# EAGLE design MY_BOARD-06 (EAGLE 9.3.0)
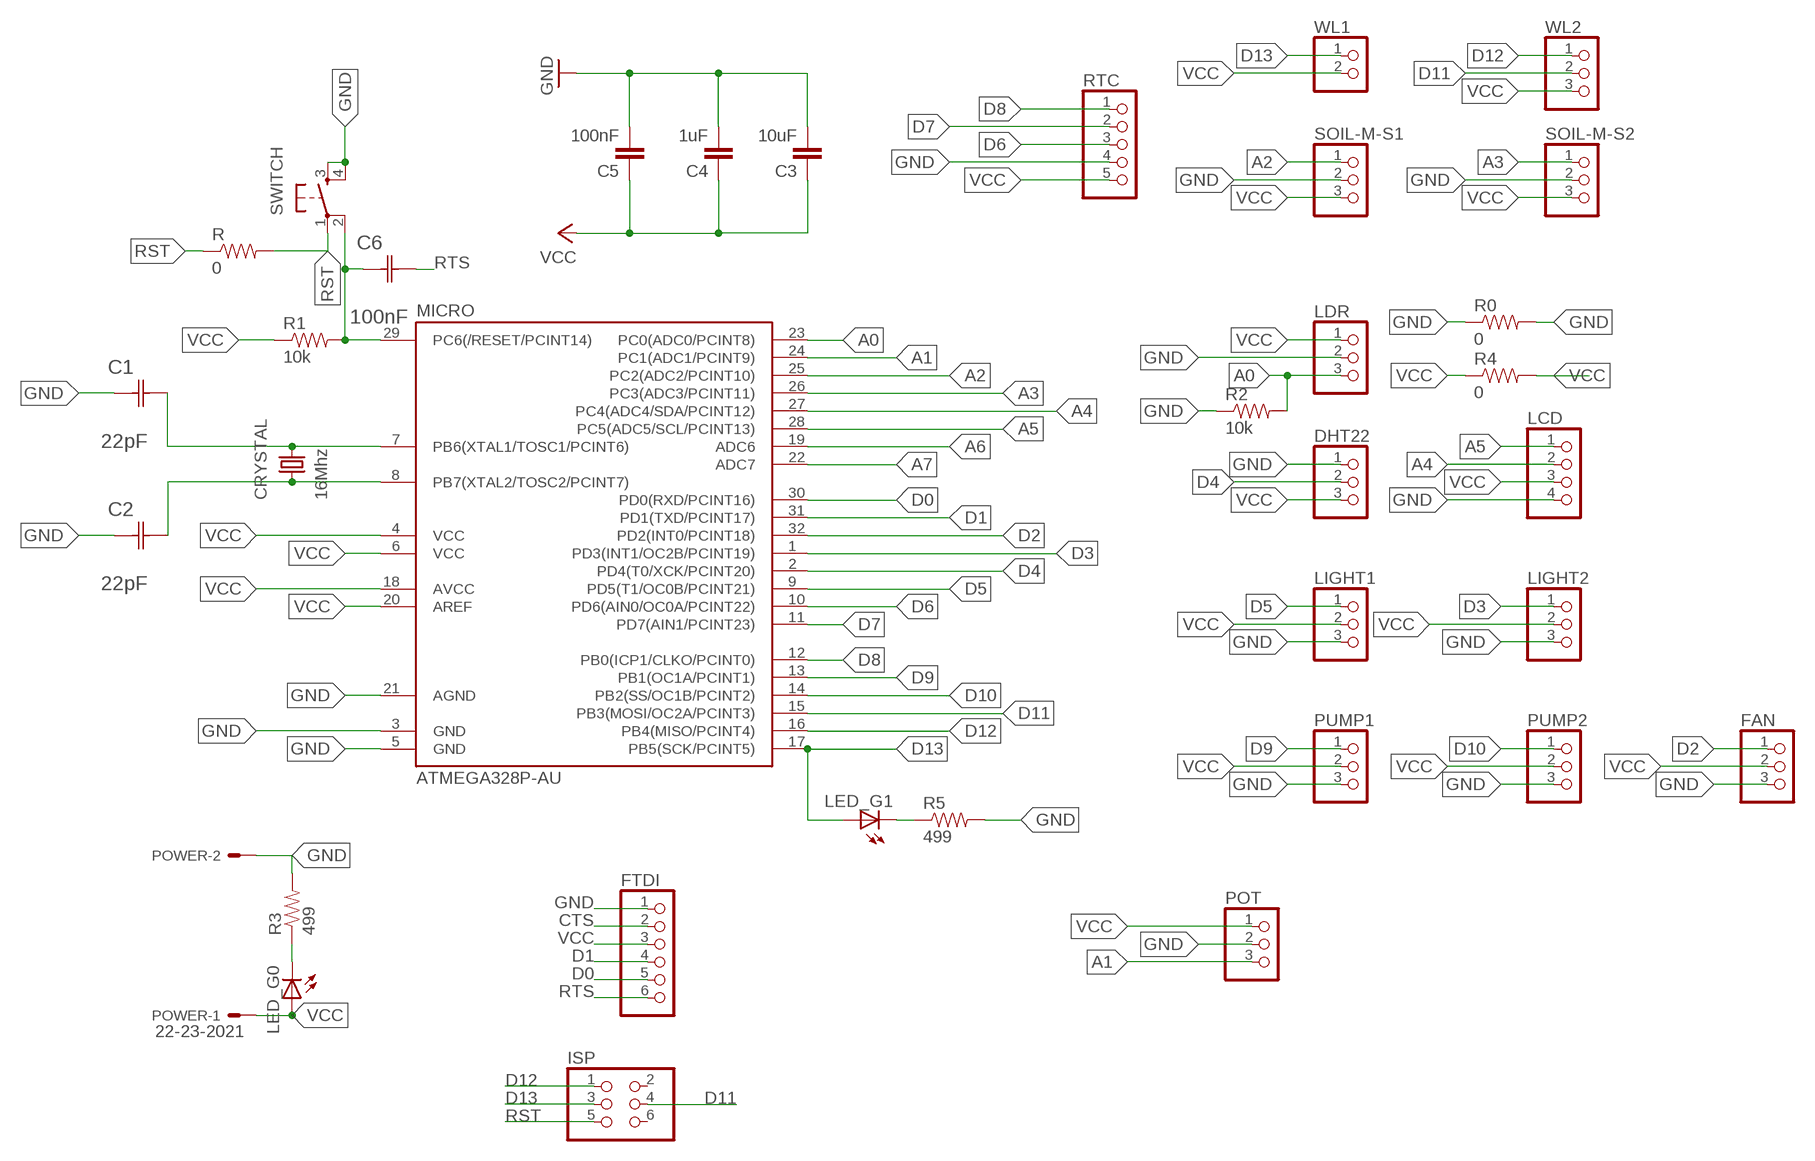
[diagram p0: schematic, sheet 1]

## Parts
C1  22pF  0612ZC225MAT2A  [CAPC3216X178N]
C2  22pF  0612ZC225MAT2A  [CAPC3216X178N]
C3  10uF  CAP1206  [1206]
C4  1uF  CAP1206  [1206]
C5  100nF  CAP1206  [1206]
C6  100nF  0612ZC225MAT2A  [CAPC3216X178N]
CRYSTAL  16Mhz  CSM-7X-DU  [CSM-7X-DU]
DHT22  PINHD-1X3/90  [1X03/90]
FAN  PINHD-1X3/90  [1X03/90]
FTDI  PINHD-1X6  [1X06]
ISP  PINHD-2X3-SMD  [2X03SMD]
LCD  PINHD-1X4/90  [1X04/90]
LDR  PINHD-1X3/90  [1X03/90]
LED_G0  LED1206  [1206]
LED_G1  LED1206  [1206]
LIGHT1  PINHD-1X3/90  [1X03/90]
LIGHT2  PINHD-1X3/90  [1X03/90]
MICRO  ATMEGA328P-AU  ATMEGA48/88/168-AU  [TQFP32-08]
POT  PINHD-1X3  [1X03]
POWER  22-23-2021  [22-23-2021]
PUMP1  PINHD-1X3/90  [1X03/90]
PUMP2  PINHD-1X3/90  [1X03/90]
R  0  RESISTOR1206  [1206]
R0  0  RESISTOR1206  [1206]
R1  10k  RESISTOR1206  [1206]
R2  10k  RESISTOR1206  [1206]
R3  499  RESISTOR1206  [1206]
R4  0  RESISTOR1206  [1206]
R5  499  RESISTOR1206  [1206]
RTC  PINHD-1X5/90  [1X05/90]
SOIL-M-S1  PINHD-1X3/90  [1X03/90]
SOIL-M-S2  PINHD-1X3/90  [1X03/90]
SWITCH  6MM_SWITCH6MM_SWITCH  [6MM_SWITCH]
WL1  PINHD-1X2/90  [1X02/90]
WL2  PINHD-1X3/90  [1X03/90]

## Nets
A0: LDR.3 MICRO.23(PC0(ADC0/PCINT8)) R2.2
A1: MICRO.24(PC1(ADC1/PCINT9)) POT.3
A2: MICRO.25(PC2(ADC2/PCINT10)) SOIL-M-S1.1
A3: MICRO.26(PC3(ADC3/PCINT11)) SOIL-M-S2.1
A4: LCD.2 MICRO.27(PC4(ADC4/SDA/PCINT12))
A5: LCD.1 MICRO.28(PC5(ADC5/SCL/PCINT13))
A6: MICRO.19(ADC6)
A7: MICRO.22(ADC7)
CTS: FTDI.2
D0: FTDI.5 MICRO.30(PD0(RXD/PCINT16))
D1: FTDI.4 MICRO.31(PD1(TXD/PCINT17))
D2: FAN.1 MICRO.32(PD2(INT0/PCINT18))
D3: LIGHT2.1 MICRO.1(PD3(INT1/OC2B/PCINT19))
D4: DHT22.2 MICRO.2(PD4(T0/XCK/PCINT20))
D5: LIGHT1.1 MICRO.9(PD5(T1/OC0B/PCINT21))
D6: MICRO.10(PD6(AIN0/OC0A/PCINT22)) RTC.3
D7: MICRO.11(PD7(AIN1/PCINT23)) RTC.2
D8: MICRO.12(PB0(ICP1/CLKO/PCINT0)) RTC.1
D9: MICRO.13(PB1(OC1A/PCINT1)) PUMP1.1
D10: MICRO.14(PB2(SS/OC1B/PCINT2)) PUMP2.1
D11: ISP.4 MICRO.15(PB3(MOSI/OC2A/PCINT3)) WL2.2
D12: ISP.1 MICRO.16(PB4(MISO/PCINT4)) WL2.1
D13: ISP.3 LED_G1.1(A) MICRO.17(PB5(SCK/PCINT5)) WL1.1
GND: C1.1(C1) C2.1(C1) C3.2 C4.2 C5.2 DHT22.1 FAN.3 FTDI.1 LCD.4 LDR.2 LIGHT1.3 LIGHT2.3 MICRO.3(GND) MICRO.5(GND) MICRO.21(AGND) POT.2 POWER.2 PUMP1.3 PUMP2.3 R0.1 R0.2 R2.1 R3.2 R5.2 RTC.4 SOIL-M-S1.2 SOIL-M-S2.2 SWITCH.3(S) SWITCH.4(S1)
LED: LED_G0.2(C) R3.1
LED1: LED_G1.2(C) R5.1
RST: C6.1(C1) ISP.5 MICRO.29(PC6(/RESET/PCINT14)) R1.2 R.1 R.2 SWITCH.1(P) SWITCH.2(P1)
RTS: C6.2(C2) FTDI.6
VCC: C3.1 C4.1 C5.1 DHT22.3 FAN.2 FTDI.3 LCD.3 LDR.1 LED_G0.1(A) LIGHT1.2 LIGHT2.2 MICRO.4(VCC) MICRO.6(VCC) MICRO.18(AVCC) MICRO.20(AREF) POT.1 POWER.1 PUMP1.2 PUMP2.2 R1.1 R4.1 R4.2 RTC.5 SOIL-M-S1.3 SOIL-M-S2.3 WL1.2 WL2.3
XTAL1: C1.2(C2) CRYSTAL.2 MICRO.7(PB6(XTAL1/TOSC1/PCINT6))
XTAL2: C2.2(C2) CRYSTAL.1 MICRO.8(PB7(XTAL2/TOSC2/PCINT7))
Unconnected: ISP.2 ISP.6

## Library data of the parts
C1 C2 C6 = AVX_By_element14_Batch_1:0612ZC225MAT2A: Capacitor 1206; MPN: 0612ZC225MAT2A; OC_FARNELL: -; OC_NEWARK: 12N3209; SUPPLIER: AVX; TOLERANCE: ±20%; VALUE: 2.2µF; VOLTAGERATING: 10V
C3-C5 = 01_SparkFun:CAP: Capacitor
CRYSTAL = 01_FAB_Hello:CSM-7X-DU: SMD CRYSTAL; OC_FARNELL: unknown; OC_NEWARK: unknown
DHT22 FAN LDR LIGHT1 LIGHT2 POT PUMP1 PUMP2 SOIL-M-S1 SOIL-M-S2 WL2 = pinhead:PINHD-1X3: PIN HEADER
FTDI = pinhead:PINHD-1X6: PIN HEADER
ISP = fab:PINHD-2X3-SMD: PIN HEADER
LCD = pinhead:PINHD-1X4: PIN HEADER
LED_G0 LED_G1 = 01_FAB_Hello:LED
MICRO = atmega8:ATMEGA48/88/168
POWER = con-molex:22-23-2021: .100" (2.54mm) Center Header - 2 Pin; MF: MOLEX; MPN: 22-23-2021; OC_FARNELL: 1462926; OC_NEWARK: 25C3832
R R0 R1-R5 = 01_SparkFun:RESISTOR: Resistor
RTC = pinhead:PINHD-1X5: PIN HEADER
SWITCH = 01_FAB_Hello:6MM_SWITCH: OMRON SWITCH
WL1 = pinhead:PINHD-1X2: PIN HEADER

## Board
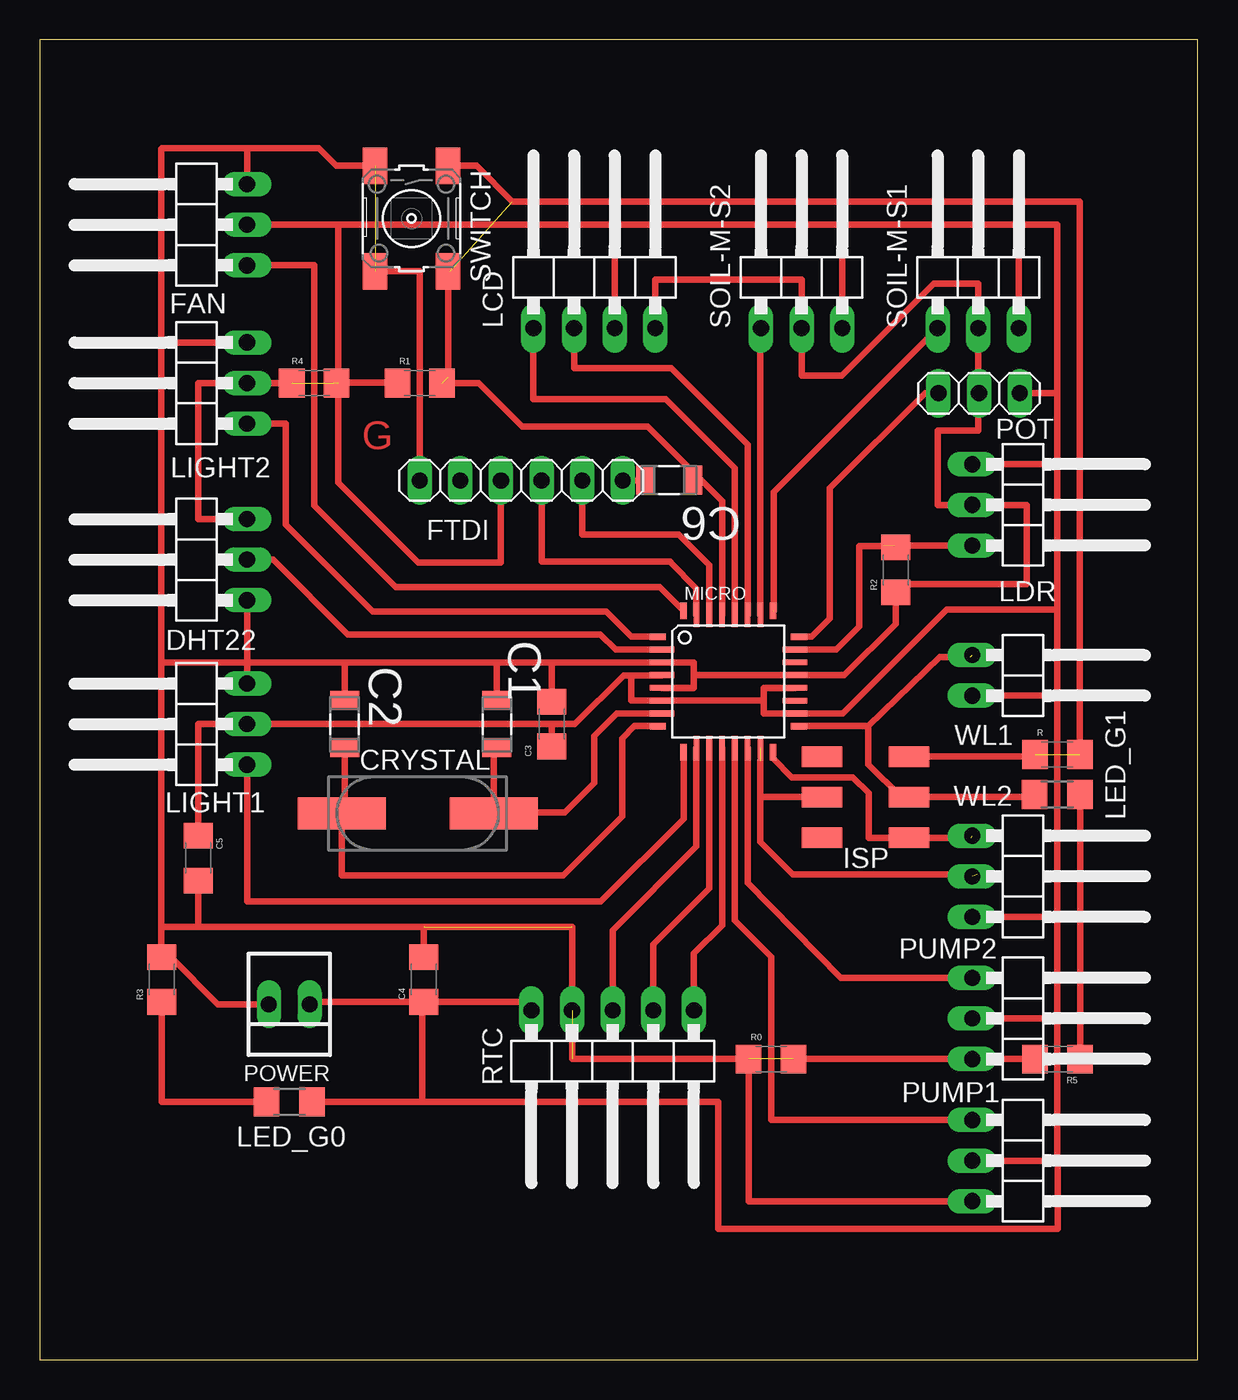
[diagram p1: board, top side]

Size 72.39 x 82.55 mm. Coordinates in mm from the lower left corner, seen from the top.
Outline: 0,0 72.39,0 72.39,82.55 0,82.55 0,0
Copper layers (1*16): Top 0.035mm / dielectric 1.5mm / Bottom 0.035mm
Design rules "default *": minimum track width 16mil, minimum drill 0.35mm, track to track 16mil, track to pad 16mil, pad to pad 16mil, via to via 16mil, smd to smd 6mil, copper to edge 40mil, drill to drill 6mil, minimum pad ring 10mil, minimum via ring 8mil, stop-mask expansion 4mil, vias tented up to drill 0mil, thermal gap 10mil

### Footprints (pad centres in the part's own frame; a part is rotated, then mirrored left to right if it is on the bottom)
CAPC3216X178N = smd 1.118 x 1.803: 1 -1.499,0; 2 1.499,0
1206 = smd 1.6 x 1.8: 1 -1.4,0; 2 1.4,0
CSM-7X-DU = smd 5.5 x 2: 1 -4.75,0; 2 4.75,0
1X03/90 = drill 1.016 long: 1 -2.54,-3.81; 2 0,-3.81; 3 2.54,-3.81
1X06 = drill 1.016 long: 1 -6.35,0; 2 -3.81,0; 3 -1.27,0; 4 1.27,0; 5 3.81,0; 6 6.35,0
2X03SMD = smd 2.54 x 1.27: 1 -2.54,2.54; 2 2.92,2.54; 3 -2.54,0; 4 2.92,0; 5 -2.54,-2.54; 6 2.92,-2.54
1X04/90 = drill 1.016 long: 1 -3.81,-3.81; 2 -1.27,-3.81; 3 1.27,-3.81; 4 3.81,-3.81
1206' = smd 1.6 x 1.803: 1 -1.422,0; 2 1.422,0
TQFP32-08 = smd 1.016 x 0.406: 1 -4.42,2.8; 8 -4.42,-2.8; 17 4.42,-2.8; 24 4.42,2.8 | smd 1.524 x 0.356: 2 -4.166,2; 3 -4.166,1.2; 4 -4.166,0.4; 5 -4.166,-0.4; 6 -4.166,-1.2; 7 -4.166,-2; 18 4.166,-2; 19 4.166,-1.2; 20 4.166,-0.4; 21 4.166,0.4; 22 4.166,1.2; 23 4.166,2 | smd 0.406 x 1.016: 9 -2.8,-4.42; 16 2.8,-4.42; 25 2.8,4.42; 32 -2.8,4.42 | smd 0.356 x 1.524: 10 -2,-4.166; 11 -1.2,-4.166; 12 -0.4,-4.166; 13 0.4,-4.166; 14 1.2,-4.166; 15 2,-4.166; 26 2,4.166; 27 1.2,4.166; 28 0.4,4.166; 29 -0.4,4.166; 30 -1.2,4.166; 31 -2,4.166
1X03 = drill 1.016 long: 1 -2.54,0; 2 0,0; 3 2.54,0
22-23-2021 = drill 1 long: 1 -1.27,0; 2 1.27,0
1X05/90 = drill 1.016 long: 1 -5.08,-3.81; 2 -2.54,-3.81; 3 0,-3.81; 4 2.54,-3.81; 5 5.08,-3.81
6MM_SWITCH = smd 2.286 x 1.524: 1 -3.302,2.286; 2 3.302,2.286; 3 -3.302,-2.286; 4 3.302,-2.286
1X02/90 = drill 1.016 long: 1 -1.27,-3.81; 2 1.27,-3.81

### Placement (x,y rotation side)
C1  28.57,39.75 270 top
C2  19.05,39.75 270 top
C3  32,39.75 90 top
C4  24,23.77 90 top
C5  9.91,31.37 270 top
C6  39.34,55.02 180 top
CRYSTAL  23.62,34.16 0 top
DHT22  9.14,50.04 90 top
FAN  9.14,70.99 90 top
FTDI  30.1,54.99 0 top
ISP  51.82,35.18 180 top
LCD  34.67,68.33 0 top
LDR  62.1,53.47 270 top
LED_G0  [1206']  15.59,16.13 180 top
LED_G1  [1206']  63.63,35.36 0 top
LIGHT1  9.14,39.75 90 top
LIGHT2  9.14,61.09 90 top
MICRO  43.05,42.42 0 top
POT  58.72,60.45 180 top
POWER  15.59,22.23 180 top
PUMP1  62.1,12.45 270 top
PUMP2  62.1,21.34 270 top
R  63.63,37.85 0 top
R0  45.72,18.8 0 top
R1  23.75,61.09 0 top
R2  53.52,49.4 90 top
R3  7.62,23.77 90 top
R4  17.14,61.09 0 top
R5  63.63,18.8 180 top
RTC  35.81,18.03 180 top
SOIL-M-S1  58.67,68.33 0 top
SOIL-M-S2  47.62,68.33 0 top
SWITCH  23.24,71.37 270 top
WL1  62.1,42.8 270 top
WL2  62.1,30.23 270 top

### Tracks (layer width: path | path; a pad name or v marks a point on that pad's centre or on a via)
A0  (1 unrouted)
  Top 0.406: 47.85,44.42 MICRO.23 49.81,44.42 51.23,45.84 51.23,50.9 53.42,50.9 R2.2 | LDR.3 52.77,50.93
A1
  Top 0.406: 47.6,45.22 MICRO.24 48.27,45.22 49.4,46.35 49.4,54.51 55.35,60.45 POT.3
A2  (1 unrouted)
  Top 0.406: SOIL-M-S1.1 45.87,54.25 45.87,46.84
A3
  Top 0.406: MICRO.26 45.05,64.48 SOIL-M-S2.1
A4
  Top 0.406: MICRO.27 44.25,57.25 39.48,62.03 33.4,62.03 LCD.2
A5
  Top 0.406: MICRO.28 43.45,55.77 39.12,60.1 30.86,60.1 LCD.1
D0
  Top 0.406: MICRO.30 41.85,49.7 39.94,51.61 33.91,51.61 FTDI.5
D1
  Top 0.406: FTDI.4 31.37,49.91 39.4,49.91 39.4,49.89 41.05,48.23 MICRO.31
D2
  Top 0.406: MICRO.32 38.76,48.34 22.25,48.34 17.14,53.42 17.14,68.45 FAN.1
D3
  Top 0.406: LIGHT2.1 15.37,58.55 15.37,52.23 20.81,46.79 35.41,46.79 36.98,45.22 MICRO.1
D4
  Top 0.406: MICRO.2 35.99,44.42 35.05,45.36 19.26,45.36 14.59,50.04 DHT22.2
D5
  Top 0.406: MICRO.9 40.25,33.83 35.07,28.65 12.95,28.65 LIGHT1.1
D6
  Top 0.406: MICRO.10 41.05,32.09 35.81,26.85 RTC.3
D7
  Top 0.406: MICRO.11 41.85,29.48 38.35,25.98 RTC.2
D8
  Top 0.406: 42.67,38.24 MICRO.12 42.65,27.16 40.89,25.4 RTC.1
D9
  Top 0.406: MICRO.13 43.45,27.46 45.72,25.2 45.72,14.99 PUMP1.1
D10
  Top 0.406: MICRO.14 44.25,29.81 50.08,23.88 PUMP2.1 58.29,23.86 PUMP2.1
D11  (2 unrouted)
  Top 0.406: 45.05,35.18 45.05,32.38 47.09,30.35 58.6,30.35 | ISP.4 45.05,35.18 | 45.05,35.18 45.05,37.45
D12  (1 unrouted)
  Top 0.406: MICRO.16 45.85,37.59 47.02,36.42 50.83,36.42 51.82,35.43 51.82,32.64 ISP.1 58.24,32.64
D13  (1 unrouted)
  Top 0.406: 58.17,43.94 56.26,43.94 51.81,39.62 51.79,39.62 | 51.79,39.62 MICRO.17 | 51.79,39.62 51.79,37.24 53.85,35.18 ISP.3 62.2,35.18 LED_G1.1
GND  (4 unrouted)
  Top 0.406: MICRO.5 40.89,42.02 40.89,42.82 | LCD.4 38.48,67.56 47.62,67.56 SOIL-M-S2.2 47.62,61.54 50.14,61.54 55.91,67.31 58.67,67.31 SOIL-M-S1.2 58.67,60.5 | 58.67,60.5 58.67,58.12 56.13,58.12 56.13,53.47 LDR.2 61.7,53.47 61.7,48.51 54.03,48.51 R2.1 53.52,46.02 50.31,42.82 MICRO.21 40.89,42.82 | R0.2 PUMP2.3 R5.2 | PUMP1.3 44.32,9.91 R0.1 33.27,18.8 33.27,27.05 29.03,27.05 9.91,27.05 | 28.57,43.62 19.05,43.62 | 19.05,43.62 12.95,43.62 | C2.1 19.05,43.62 | C1.1 28.57,43.62 | LIGHT1.3 12.95,43.62 | DHT22.1 12.95,43.62 | 32,43.62 MICRO.3 40.89,43.62 40.89,42.82 | 32,43.62 28.57,43.62 | 32,43.62 C3.2 | 23.9,27.05 24,27.05 C4.2 | 9.91,27.05 7.57,27.05 | 7.57,27.05 7.57,43.62 | 7.57,43.62 12.95,43.62 | 7.57,43.62 7.57,63.65 | 7.57,63.65 7.57,75.74 7.62,75.79 12.95,75.79 | C5.2 9.91,27.05 | SWITCH.4 23.75,68.07 FTDI.1 | SWITCH.3 18.54,74.68 17.42,75.79 12.95,75.79 | 7.57,27.05 7.57,25.23 R3.2 8.18,25.17 11.13,22.23 POWER.2 | 7.57,63.65 7.59,63.63 LIGHT2.3 | FAN.3 12.95,75.79 | POT.2 58.67,60.5
LED
  Top 0.406: LED_G0.2 7.62,16.13 R3.1
LED1
  Top 0.406: R5.1 65.05,19.14 LED_G1.2
RST  (3 unrouted)
  Top 0.406: MICRO.29 42.65,53.71 41.11,55.26 | 25.65,68.07 SWITCH.2 | SWITCH.2 25.2,67.75 | 41.11,55.26 37.99,58.37 30.15,58.37 27.43,61.09 R1.2 | SWITCH.2 25.53,61.46 | ISP.5 62.23,37.72 R.1 | R.2 65.03,72.44 29.54,72.44 27.3,74.68 SWITCH.1 | C6.1 40.87,55.02 41.11,55.26
RTS
  Top 0.406: FTDI.6 37.82,54.99 C6.2
VCC  (5 unrouted)
  Top 0.406: 47.23,42 MICRO.20 45.26,42.02 45.26,41.22 | 38.9,41.23 MICRO.6 | 63.63,41.53 63.63,27.74 | 63.63,27.74 63.5,27.69 | 63.63,27.74 63.5,27.69 | 63.5,27.69 WL2.3 | WL1.2 63.63,41.53 | SOIL-M-S2.3 50.16,70.99 | 61.21,70.99 63.62,70.99 63.62,60.43 | 61.21,70.99 50.16,70.99 | 63.63,41.53 63.63,46.93 | 63.63,21.34 PUMP2.2 | 63.63,27.74 63.63,21.34 | 63.63,12.45 63.65,12.45 63.65,8.18 42.42,8.18 42.42,16.13 23.9,16.13 | 63.63,12.45 PUMP1.2 | 63.63,21.34 63.63,12.45 | 63.63,46.93 56.71,46.93 50.2,40.42 MICRO.18 45.26,40.42 45.26,41.22 | LDR.1 63.63,56.01 63.63,46.93 | 63.62,55.95 63.62,60.43 | 50.16,70.99 35.94,70.99 | 35.94,70.99 LCD.3 | 22.48,61.22 R1.1 22.32,61.11 18.64,61.11 18.64,54.88 23.66,49.86 28.83,49.86 FTDI.3 | DHT22.3 9.91,52.58 9.91,61.09 LIGHT2.2 R4.1 | MICRO.4 38.89,42.8 36.98,42.8 | 36.98,42.8 36.5,42.8 33.45,39.75 32,39.75 | 32.64,38.57 32.64,38.73 C3.1 32,39.75 | C5.1 9.91,39.75 LIGHT1.2 32,39.75 | MICRO.6 45.26,41.22 | SOIL-M-S1.3 61.21,70.99 | 18.64,61.09 18.64,70.99 | 18.64,70.99 35.94,70.99 | LED_G0.1 23.9,16.13 | C4.1 30.2,22.37 RTC.5 | C4.1 23.9,22.28 23.9,16.13 | C4.1 17.01,22.37 POWER.1 | 18.39,61.11 18.36,61.09 | 18.64,70.99 FAN.2 | POT.1 63.59,60.45 63.62,60.43 | MICRO.6 36.98,41.22 36.98,42.8
XTAL1
  Top 0.406: C1.2 28.37,38.43 CRYSTAL.2 28.37,34.21 32.82,34.21 34.67,36.07 34.67,39.01 36.08,40.42 MICRO.7
XTAL2
  Top 0.406: C2.2 19.05,34.16 CRYSTAL.1 18.87,30.28 32.72,30.28 36.4,33.96 36.4,38.86 37.16,39.62 MICRO.8

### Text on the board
Top: G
